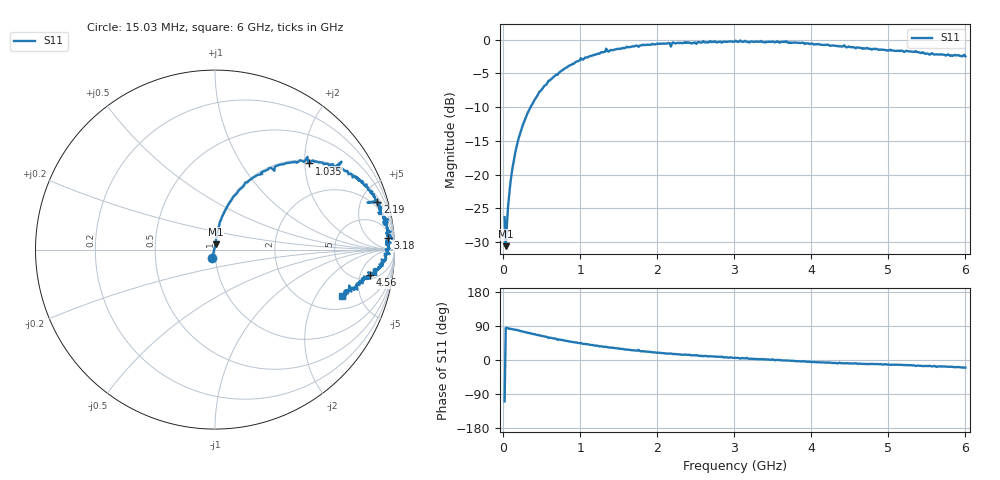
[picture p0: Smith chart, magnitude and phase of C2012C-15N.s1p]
!	Network	Analyzer	HP8753E.07.74:	Oct	30	2002	Serial	No.	JP38451487
!	Hewlett-Packard
!	7	Sep	2009	10:45:36
!	Frequency	S11
#	HZ	S	RI	R	50
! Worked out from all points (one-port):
!   400 points, 15.03 MHz to 6 GHz, reference 50 ohm
!   lowest |S11| = -30.6 dB at 30.03 MHz (marker M1), VSWR 1.06, Z = 50.2 + j2.94 ohm
!   |S11| at or under -10 dB: start of sweep to 352.5 MHz
!   S11 on the Smith chart (normalised r, x): 15.03 MHz: 0.96, -0.09; 1.035 GHz: 1.08, +2.11; 2.19 GHz: 1.41, +6.71; 3.18 GHz: 12, +23; 4.56 GHz: 6.04, -7.35; 6 GHz: 2.82, -3.40
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1.502992e7  -0.0158 -0.0457
3.002985e7  0.00282 0.0293
6.00297e7  0.00622 0.0578
1.050295e8  0.0147 0.0994
1.650292e8  0.0273 0.154
2.550287e8  0.0618 0.228
4.650277e8  0.17 0.375
7.650262e8  0.358 0.472
1.005025e9  0.515 0.517
1.035025e9  0.526 0.48
1.335023e9  0.705 0.49
1.365023e9  0.683 0.447
1.515022e9  0.743 0.42
1.725021e9  0.823 0.38
1.755021e9  0.79 0.401
1.785021e9  0.838 0.353
1.93502e9  0.876 0.321
2.145019e9  0.905 0.275
2.175019e9  0.85 0.262
2.190019e9  0.905 0.264
2.265019e9  0.916 0.249
3.015015e9  0.979 0.0998
3.180014e9  0.963 0.0653
3.765011e9  0.949 -0.0341
4.515007e9  0.873 -0.137
4.560007e9  0.864 -0.142
5.265004e9  0.798 -0.195
6e9  0.708 -0.26
